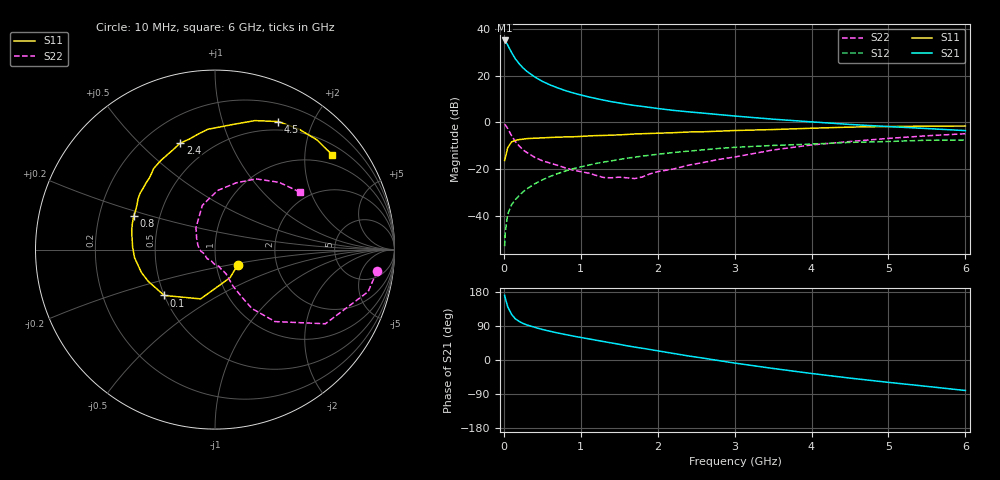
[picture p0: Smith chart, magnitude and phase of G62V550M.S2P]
! SIEMENS Small Signal Semiconductors
! BFG193
! Si NPN RF Bipolar Junction Transistor in SOT223
! VCE = 2.5 V  IC = 50 mA
! Common Emitter S-Parameters:  August  1996
# GHz  S  MA  R  50
!  f  S11  S21  S12  S22
! GHz  MAG  ANG  MAG  ANG  MAG  ANG  MAG  ANG
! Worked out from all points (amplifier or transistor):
!   36 points, 10 MHz to 6 GHz, reference 50 ohm
!   highest |S21| = 35.2 dB at 10 MHz (marker M1)
!   |S21| within 3 dB of that: start of sweep to 66.3 MHz
!   unconditionally stable (mu >= 1): 391.7 MHz to 2.398 GHz
!   at 250 MHz: K = 0.93, MSG = 26.6 dB, |S12| = -29.8 dB
!   at 1.4 GHz: K = 1.05, MAG = 11.3 dB, |S12| = -16.5 dB
!   at 6 GHz: K = 0.92, MSG = 2.0 dB, |S12| = -7.6 dB
!   S11 on the Smith chart (normalised r, x): 10 MHz: 1.26, -0.22; 100 MHz: 0.50, -0.30; 800 MHz: 0.35, +0.17; 2.4 GHz: 0.34, +0.67; 4.5 GHz: 0.40, +1.54; 6 GHz: 0.74, +2.65
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0.01  0.1525 -34.7  57.84 170.5  0.0022 84.8  0.9109 -7.6
0.02  0.1776 -61.7  55.52 162.3  0.0046 78.7  0.8845 -15.4
0.05  0.2861 -106.3  46.16 140.6  0.0107 71.8  0.7408 -33.9
0.1  0.3812 -137.9  31.96 120.6  0.017 67.4  0.5219 -50.2
0.15  0.4123 -154.7  23.23 108.5  0.0221 65.7  0.3877 -57.9
0.2  0.4294 -162.8  18.24 101.7  0.027 68.0  0.3126 -60.2
0.25  0.4386 -169.1  14.86 96.5  0.0324 67.5  0.2575 -62.3
0.3  0.4506 -174.3  12.53 92.5  0.0374 68.9  0.226 -63.7
0.4  0.4591 178.3  9.539 86.4  0.0479 68.8  0.1788 -64.7
0.5  0.4668 171.9  7.659 80.6  0.0583 67.7  0.1505 -65.4
0.6  0.476 167.1  6.427 75.9  0.0692 67.1  0.1342 -67.5
0.7  0.483 162.4  5.532 71.3  0.0798 65.6  0.1199 -71.1
0.8  0.4896 157.7  4.835 67.2  0.0905 63.9  0.1056 -74.4
1.1  0.5136 146.6  3.545 55.9  0.121 58.4  0.0818 -92.0
1.3  0.5267 139.4  3.013 48.5  0.1415 54.1  0.0656 -108.7
1.6  0.5532 129.6  2.454 37.6  0.1706 47.2  0.0647 -141.5
2.2  0.6026 113.0  1.823 17.5  0.2259 33.2  0.0997 164.0
2.4  0.624 108.1  1.692 10.7  0.2421 29.0  0.1209 148.1
3.5  0.7045 81.8  1.177 -22.3  0.3212 1.5  0.2567 105.9
4.5  0.7957 63.7  0.907 -47.8  0.3733 -18.5  0.3903 72.4
5.5  0.8345 47.1  0.741 -69.6  0.415 -41.7  0.5176 46.4
6  0.8399 38.9  0.669 -80.5  0.4188 -55.0  0.5727 33.9
